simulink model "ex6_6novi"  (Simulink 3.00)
settings: Solver=ode15s  SolverMode=SingleTasking  StartTime=0.0  StopTime=1000  RelTol=1e-3  AbsTol=1e-6

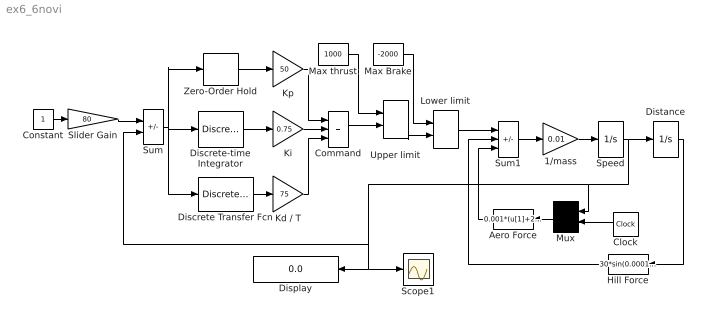
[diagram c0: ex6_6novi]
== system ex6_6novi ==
  1/mass : Gain  Gain=0.01  SaturateOnIntegerOverflow=on
  Aero Force : Fcn  Orientation=left  Expr=0.001*(u[1]+20*sin(0.01*u[2]))^2
  Clock : Clock
  Command : Sum  Inputs=+++  SaturateOnIntegerOverflow=on
  Constant : Constant  Value=1
  Discrete Transfer Fcn : DiscreteTransferFcn  Numerator=[1 -1]  Denominator=[1 0]  SampleTime=0.5
  Discrete-time Integrator : DiscreteIntegrator  IntegratorMethod=ForwardEuler  ExternalReset=none  InitialConditionSource=internal  InitialCondition=0  LimitOutput=on  UpperSaturationLimit=100  LowerSaturationLimit=-100  ShowSaturationPort=off  ShowStatePort=off  SampleTime=0.5
  Display : Display
  Distance : Integrator  ExternalReset=none  InitialConditionSource=internal  InitialCondition=0  LimitOutput=off  UpperSaturationLimit=inf  LowerSaturationLimit=-inf  ShowSaturationPort=off  ShowStatePort=off  AbsoluteTolerance=auto
  Hill Force : Fcn  Orientation=left  Expr=30*sin(0.0001*u[1])
  Kd / T : Gain  Gain=75  SaturateOnIntegerOverflow=on
  Ki : Gain  Gain=0.75  SaturateOnIntegerOverflow=on
  Kp : Gain  Gain=50  SaturateOnIntegerOverflow=on
  Lower limit : MinMax  Function=max  Inputs=2
  Max Brake : Constant  Value=-2000
  Max thrust : Constant  Value=1000
  Mux : Mux  Orientation=left  Inputs=2
  Scope1 : Scope
  Slider Gain : Gain  LoadFcn=slideg Load  Gain=80  SaturateOnIntegerOverflow=on  mask(Slider Gain){}
  Speed : Integrator  ExternalReset=none  InitialConditionSource=internal  InitialCondition=0  LimitOutput=off  UpperSaturationLimit=inf  LowerSaturationLimit=-inf  ShowSaturationPort=off  ShowStatePort=off  AbsoluteTolerance=auto
  Sum : Sum  Inputs=+-  SaturateOnIntegerOverflow=on
  Sum1 : Sum  Inputs=+--  SaturateOnIntegerOverflow=on
  Upper limit : MinMax  Function=min  Inputs=2
  Zero-Order Hold : ZeroOrderHold  SampleTime=0.5
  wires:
  Speed/1 -> Distance/1, Scope1/1, Display/1, Sum/2, Mux/1
  Clock/1 -> Mux/2
  Lower limit/1 -> Sum1/1
  Max Brake/1 -> Lower limit/1
  Max thrust/1 -> Upper limit/1
  Upper limit/1 -> Lower limit/2
  1/mass/1 -> Speed/1
  Sum1/1 -> 1/mass/1
  Distance/1 -> Hill Force/1
  Hill Force/1 -> Sum1/2
  Aero Force/1 -> Sum1/3
  Mux/1 -> Aero Force/1
  Constant/1 -> Slider Gain/1
  Slider Gain/1 -> Sum/1
  Zero-Order Hold/1 -> Kp/1
  Discrete-time Integrator/1 -> Ki/1
  Sum/1 -> Discrete-time Integrator/1, Zero-Order Hold/1, Discrete Transfer Fcn/1
  Discrete Transfer Fcn/1 -> Kd / T/1
  Kp/1 -> Command/1
  Ki/1 -> Command/2
  Kd / T/1 -> Command/3
  Command/1 -> Upper limit/2
